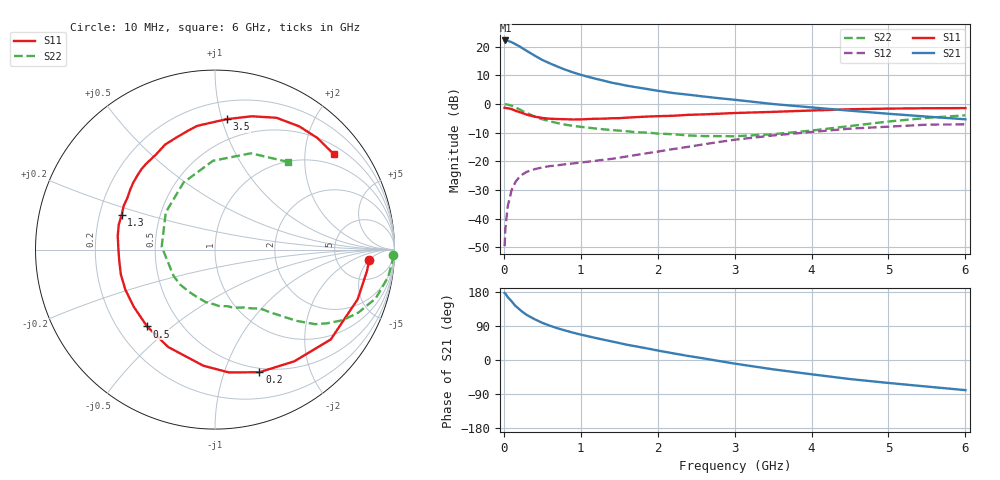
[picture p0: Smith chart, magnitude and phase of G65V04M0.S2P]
! SIEMENS Small Signal Semiconductors
! BFG193
! Si NPN RF Bipolar Junction Transistor in SOT223
! VCE = 5 V  IC = 4 mA
! Common Emitter S-Parameters:  August  1996
# GHz  S  MA  R  50
!  f  S11  S21  S12  S22
! GHz  MAG  ANG  MAG  ANG  MAG  ANG  MAG  ANG
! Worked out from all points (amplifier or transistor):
!   36 points, 10 MHz to 6 GHz, reference 50 ohm
!   highest |S21| = 22.2 dB at 20 MHz (marker M1)
!   |S21| within 3 dB of that: start of sweep to 258.9 MHz
!   unconditionally stable (mu >= 1): 1.206 GHz to 2.49 GHz
!   at 250 MHz: K = 0.28, MSG = 21.9 dB, |S12| = -24.5 dB
!   at 1.4 GHz: K = 1.08, MAG = 11.6 dB, |S12| = -19.1 dB
!   at 6 GHz: K = 0.88, MSG = 0.9 dB, |S12| = -7.1 dB
!   S11 on the Smith chart (normalised r, x): 10 MHz: 11, -5; 200 MHz: 0.46, -1.32; 500 MHz: 0.32, -0.41; 1.3 GHz: 0.29, +0.16; 3.5 GHz: 0.33, +1.04; 6 GHz: 0.70, +2.67
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0.01  0.8606 -4.0  12.83 177.0  0.0033 94.6  0.9933 -1.8
0.02  0.8553 -8.0  12.87 175.4  0.0066 85.4  0.9902 -3.6
0.05  0.8416 -19.2  12.68 166.1  0.0162 79.1  0.9773 -8.9
0.1  0.8164 -37.8  12.04 155.1  0.0312 71.3  0.9355 -16.9
0.15  0.7635 -54.6  11.1 143.0  0.0434 62.2  0.8718 -23.8
0.2  0.7265 -70.1  10.22 134.2  0.0529 56.2  0.8118 -29.0
0.25  0.6889 -83.5  9.268 125.8  0.0599 50.6  0.7463 -33.4
0.3  0.6504 -95.7  8.424 118.6  0.0657 46.9  0.6951 -36.7
0.4  0.6021 -115.7  7.011 107.7  0.0729 41.2  0.6041 -41.1
0.5  0.5715 -131.5  5.874 98.0  0.0782 37.3  0.5415 -44.0
0.6  0.5534 -145.0  5.111 90.4  0.0825 35.7  0.4986 -46.4
0.7  0.5471 -156.0  4.488 83.6  0.0852 34.6  0.4645 -48.8
0.9  0.537 -174.0  3.565 72.1  0.0918 34.2  0.4151 -52.5
1.1  0.5472 172.0  2.972 62.4  0.0986 34.8  0.3858 -58.0
1.3  0.5546 159.6  2.55 53.4  0.1066 35.9  0.3611 -63.2
1.6  0.5785 144.7  2.088 40.3  0.1217 36.7  0.3345 -73.9
2.2  0.6236 121.8  1.556 17.7  0.1635 34.3  0.2971 -100.1
2.8  0.6771 103.4  1.262 -2.8  0.2176 26.9  0.2749 -134.6
3.5  0.7297 84.9  1 -24.6  0.2825 12.5  0.2974 176.8
4.5  0.8104 65.0  0.765 -50.3  0.3721 -8.8  0.4128 115.1
5.5  0.8439 47.5  0.603 -70.1  0.4362 -35.8  0.5728 69.5
6  0.8489 38.9  0.541 -79.5  0.4423 -50.8  0.6348 50.4
